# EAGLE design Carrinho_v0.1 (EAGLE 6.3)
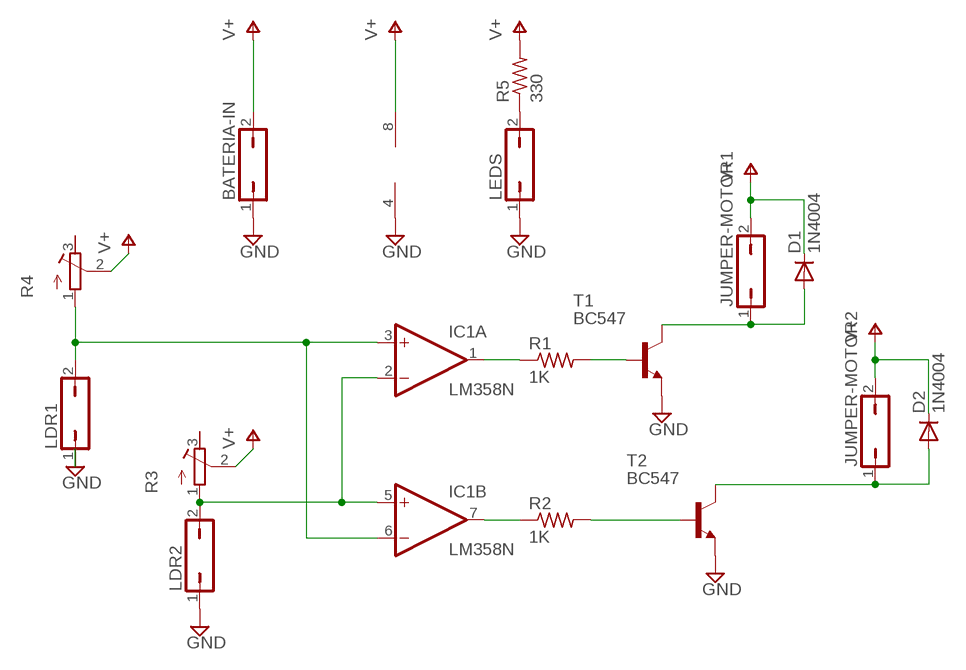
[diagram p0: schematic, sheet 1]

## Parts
BATERIA-IN  JP1Q  [JP1]
D1  1N4004  [DO41-10]
D2  1N4004  [DO41-10]
IC1  LM358N  [DIL08]
JUMPER-MOTOR1  JP1Q  [JP1]
JUMPER-MOTOR2  JP1Q  [JP1]
LDR1  JP1Q  [JP1]
LDR2  JP1Q  [JP1]
LEDS  JP1Q  [JP1]
R1  1K  R-US_0207/12  [0207/12]
R2  1K  R-US_0207/12  [0207/12]
R3  R-TRIMM64W  [RTRIM64W]
R4  R-TRIMM64W  [RTRIM64W]
R5  330  R-US_0207/12  [0207/12]
T1  BC547  [TO92]
T2  BC547  [TO92]

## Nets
N$1: IC1.7(B:OUT) R2.1
N$2: R2.2 T2.2(B)
N$3: R1.2 T1.2(B)
N$4: IC1.1(A:OUT) R1.1
N$5: IC1.3(A:+IN) IC1.6(B:-IN) LDR1.2 R4.1(A)
N$6: IC1.2(A:-IN) IC1.5(B:+IN) LDR2.2 R3.1(A)
N$7: D2.A JUMPER-MOTOR2.1 T2.3(C)
N$8: D1.A JUMPER-MOTOR1.1 T1.3(C)
N$9: LEDS.2 R5.1
N$18: BATERIA-IN.1 IC1.4(P:V-) LDR1.1 LDR2.1 LEDS.1 T1.1(E) T2.1(E) ; supply symbol labelled GND
V+: BATERIA-IN.2 D1.C D2.C IC1.8(P:V+) JUMPER-MOTOR1.2 JUMPER-MOTOR2.2 R3.2(S) R4.2(S) R5.2
Unconnected: R3.3(E) R4.3(E)

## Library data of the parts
BATERIA-IN JUMPER-MOTOR1 JUMPER-MOTOR2 LDR1 LDR2 LEDS = jumper:JP1Q: JUMPER
D1 D2 = diode:1N4004: DIODE
IC1 = linear:LM358: OP AMP also LM158; LM258; LM2904 Source: http://cache.national.com/ds/LM/LM158.pdf
R1 R2 R5 = resistor:R-US_: RESISTOR, American symbol
R3 R4 = rcl:R-TRIMM: Trimm resistor
T1 T2 = transistor:BC547: NPN TRANSISTOR

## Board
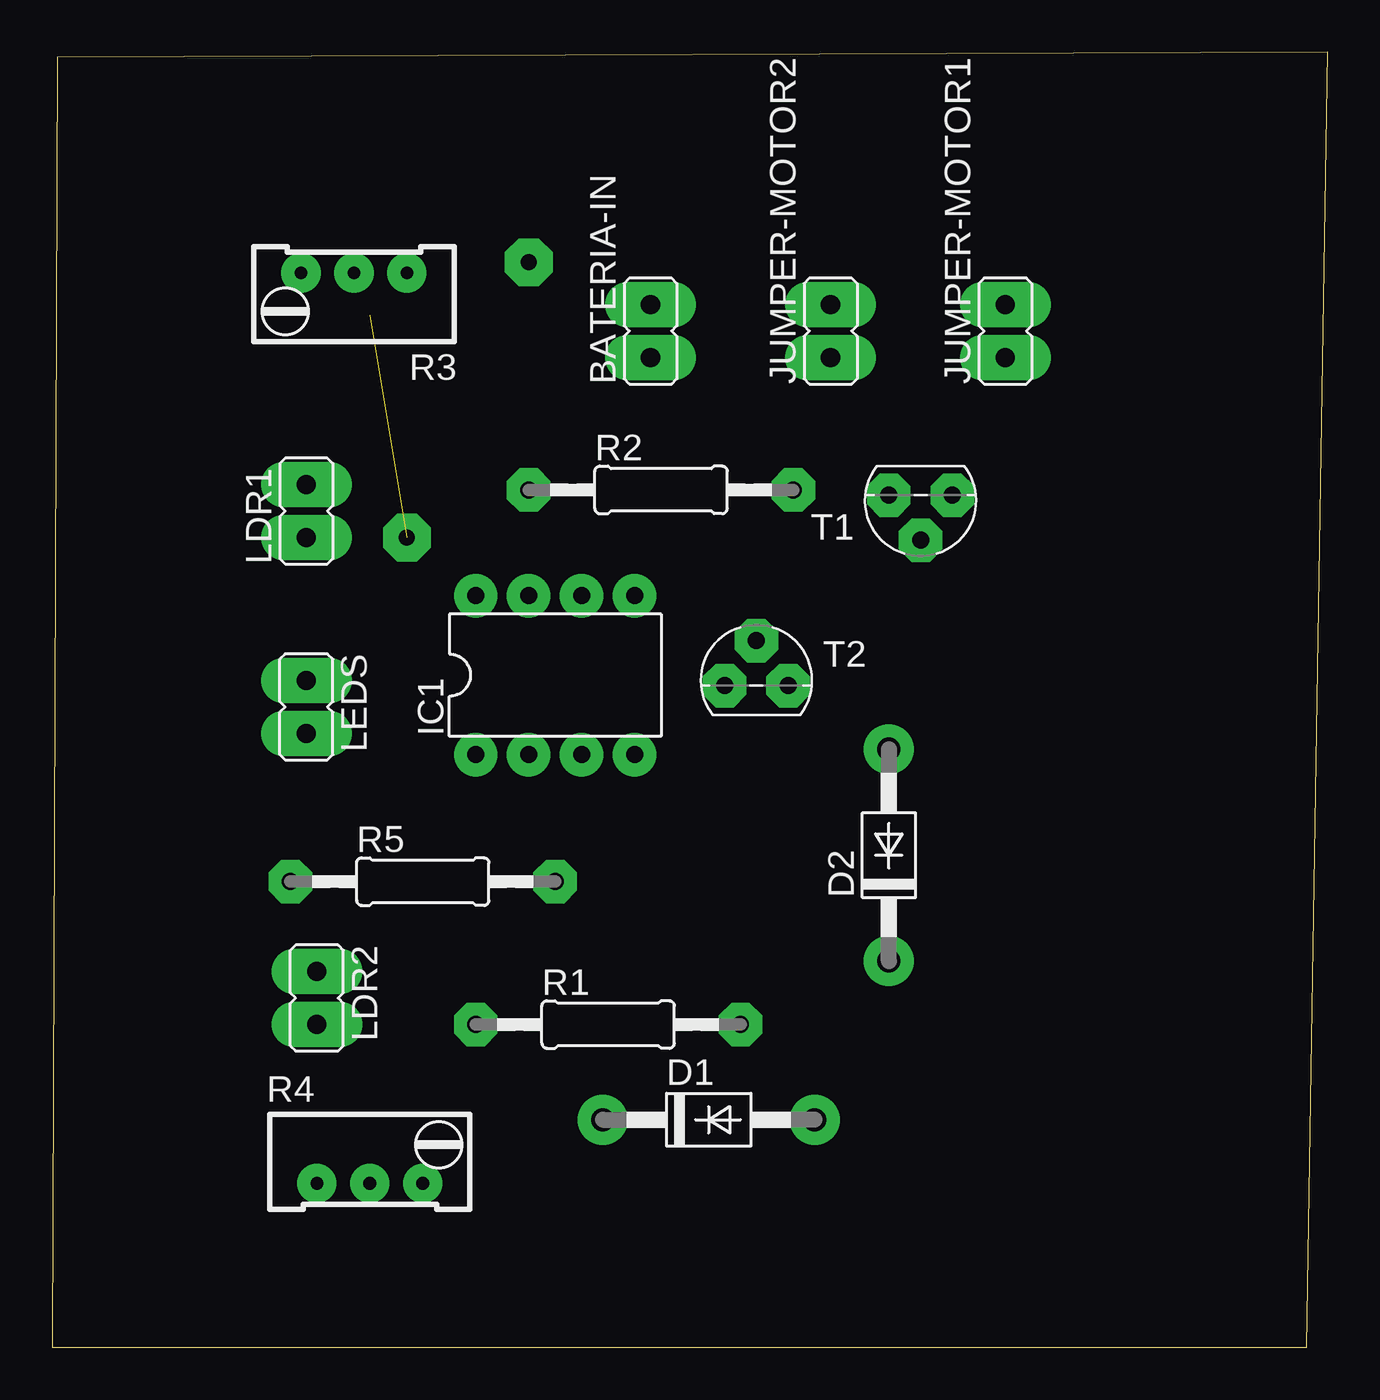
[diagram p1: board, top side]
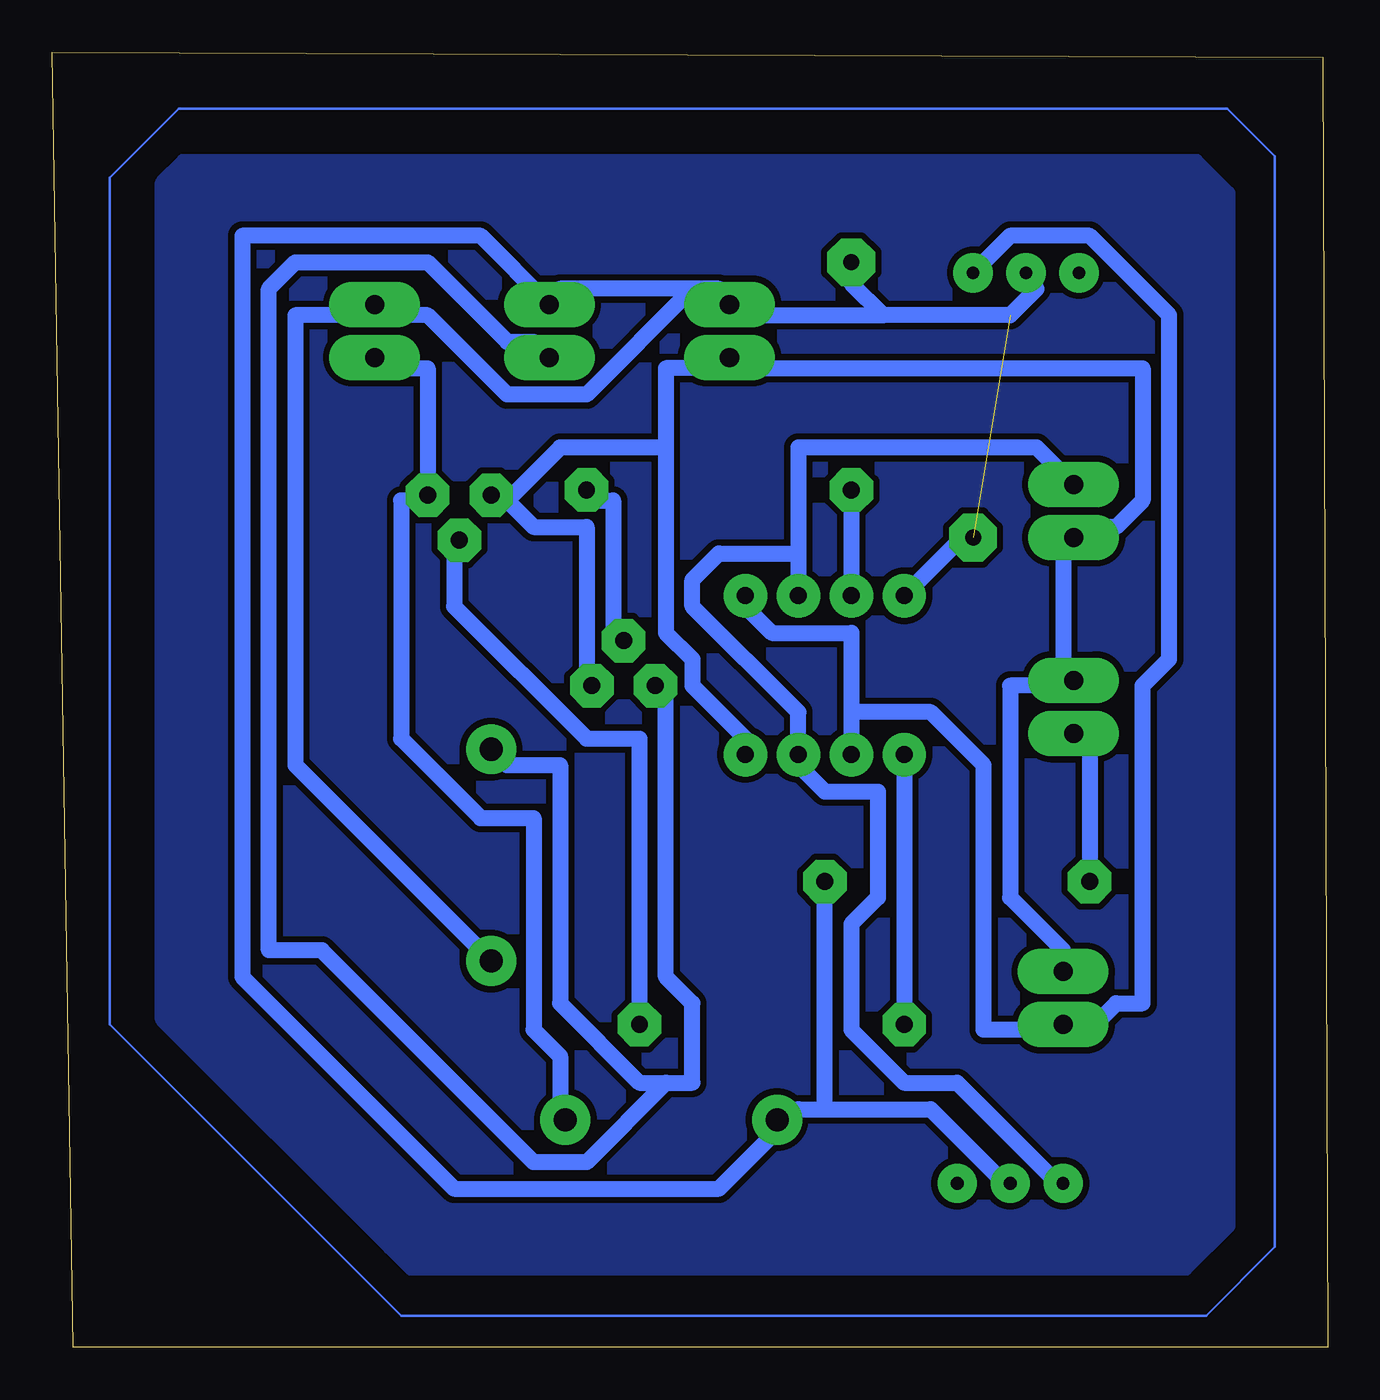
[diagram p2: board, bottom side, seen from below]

Size 61.19 x 62.15 mm. Coordinates in mm from the lower left corner, seen from the top.
Outline: 0,0 60.18,0 61.19,62.15 0.25,61.9 0,0
Copper layers (1*16): Top 0.035mm / dielectric 1.5mm / Bottom 0.035mm
Design rules "default *": minimum track width 30mil, minimum drill 24mil, track to track 12mil, track to pad 12mil, pad to pad 12mil, via to via 12mil, smd to smd 8mil, copper to edge 40mil, drill to drill 12mil, minimum pad ring 25mil, minimum via ring 30mil, stop-mask expansion 4mil, vias tented up to drill 0mil, thermal gap 10mil

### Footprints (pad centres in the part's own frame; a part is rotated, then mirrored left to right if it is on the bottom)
JP1 = drill 0.914 long: 1 0,-1.27; 2 0,1.27
DO41-10 = drill 1.118: A 5.08,0; C -5.08,0
DIL08 = drill 0.813 pad 1.27: 1 -3.81,-3.81; 2 -1.27,-3.81; 3 1.27,-3.81; 4 3.81,-3.81; 5 3.81,3.81; 6 1.27,3.81; 7 -1.27,3.81; 8 -3.81,3.81
0207/12 = drill 0.813 octagon: 1 -6.35,0; 2 6.35,0
RTRIM64W = drill 0.61: 1 1.27,-2.54; 2 1.27,0; 3 1.27,2.54
TO92 = drill 0.813 octagon: 1 1.524,-0.254; 2 0,1.905; 3 -1.524,-0.254

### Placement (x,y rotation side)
BATERIA-IN  28.7,48.77 0 top
D1  31.5,10.92 0 top
D2  40.13,23.62 90 top
IC1  24.13,32.26 0 top
JUMPER-MOTOR1  45.72,48.77 0 top
JUMPER-MOTOR2  37.34,48.77 0 top
LDR1  12.19,40.13 0 top
LDR2  12.7,16.76 180 top
LEDS  12.19,30.73 180 top
R1  26.67,15.49 0 top
R2  29.21,41.15 0 top
R3  14.48,50.29 90 top
R4  15.24,9.14 270 top
R5  17.78,22.35 0 top
T1  41.66,40.64 180 top
T2  33.78,32 0 top

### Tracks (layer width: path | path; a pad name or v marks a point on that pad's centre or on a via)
N$1
  Bottom 0.762: R2.1 IC1.7
N$2
  Bottom 0.762: T2.2 34.29,34.29 34.29,40.64 35.56,40.64 R2.2
N$3
  Bottom 0.762: R1.2 33.02,29.21 35.56,29.21 41.91,35.56 41.91,38.1 T1.2
N$4
  Bottom 0.762: IC1.1 R1.1
N$5
  Bottom 0.762: 25.4,38.1 25.4,43.18 13.97,43.18 LDR1.2 | 25.4,38.1 IC1.6 | R4.1 12.7,7.62 17.78,12.7 20.32,12.7 22.86,15.24 22.86,20.32 21.59,21.59 21.59,26.67 24.13,26.67 25.4,27.94 IC1.3 25.4,30.48 30.48,35.56 30.48,36.83 29.21,38.1 25.4,38.1
N$6
  Bottom 0.762: 22.86,30.48 22.86,34.29 26.67,34.29 27.94,35.56 IC1.5 | 22.86,30.48 IC1.2 | R3.1 15.24,53.34 11.43,53.34 7.62,49.53 7.62,33.02 8.89,31.75 8.89,16.51 10.16,16.51 11.43,15.24 12.7,15.24 | 22.86,30.48 19.05,30.48 16.51,27.94 16.51,15.24 12.7,15.24 | 12.7,15.24 LDR2.2
N$7
  Bottom 0.762: 31.75,12.7 33.02,12.7 36.83,16.51 36.83,27.94 39.37,27.94 D2.A | 31.75,12.7 30.48,12.7 30.48,16.51 31.75,17.78 31.75,31.75 T2.3 | 31.75,12.7 35.56,8.89 38.1,8.89 48.26,19.05 50.8,19.05 50.8,50.8 49.53,52.07 43.18,52.07 39.37,48.26 38.1,48.26 JUMPER-MOTOR2.1
N$8
  Bottom 0.762: JUMPER-MOTOR1.1 45.72,46.99 43.18,46.99 T1.3 43.18,40.64 44.45,40.64 44.45,29.21 40.64,25.4 38.1,25.4 38.1,15.24 36.83,13.97 36.83,11.43 D1.A
N$9
  Bottom 0.762: R5.1 11.43,29.21 LEDS.2
N$10  (via drill 0.76)
  other vias: 22.86,52.07
N$11  (via drill 0.76)
  other vias: 17.02,38.86
N$12
  pour Bottom: 4.83,55.37 4.83,6.35 4.83,5.84 6.86,3.81 43.94,3.81 44.96,4.83 55.88,15.75 55.88,55.88 54.86,56.9 6.35,56.9
N$13
  Bottom 0.127: 2.54,57.15 2.54,4.83 5.84,1.52 44.45,1.52 58.42,15.49 58.42,56.13 55.12,59.44 4.83,59.44 2.54,57.15
N$18
  Bottom 0.762: LDR2.1 12.7,19.05 15.24,21.59 15.24,31.75 12.7,31.75 LEDS.1 12.7,33.02 12.7,38.1 LDR1.1 11.43,39.37 10.16,39.37 8.89,40.64 8.89,46.99 27.94,46.99 BATERIA-IN.1 29.21,46.99 31.75,46.99 31.75,43.18 | 39.37,40.64 38.1,39.37 35.56,39.37 35.56,31.75 T2.1 | 31.75,43.18 31.75,34.29 30.48,33.02 30.48,31.75 27.94,29.21 IC1.4 | 39.37,40.64 36.83,43.18 31.75,43.18 | 39.37,40.64 T1.1
V+  (1 unrouted)
  Bottom 0.762: 24.13,11.43 25.4,11.43 D1.C 26.67,10.16 29.21,7.62 41.91,7.62 52.07,17.78 52.07,53.34 40.64,53.34 JUMPER-MOTOR2.2 36.83,50.8 30.48,50.8 | 24.13,11.43 19.05,11.43 15.24,7.62 R4.2 | 24.13,11.43 R5.2 | 21.34,49.53 27.94,49.53 BATERIA-IN.2 | R3.2 13.97,50.8 15.24,49.53 21.34,49.53 | 30.48,50.8 29.21,50.8 BATERIA-IN.2 | 45.72,49.53 43.18,49.53 39.37,45.72 35.56,45.72 30.48,50.8 | 30.48,50.8 BATERIA-IN.2 | D2.C 49.53,27.94 49.53,49.53 45.72,49.53 | 45.72,49.53 JUMPER-MOTOR1.2 | IC1.8 17.53,38.86 17.02,38.86 | 21.34,49.53 22.86,51.05 22.86,52.07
